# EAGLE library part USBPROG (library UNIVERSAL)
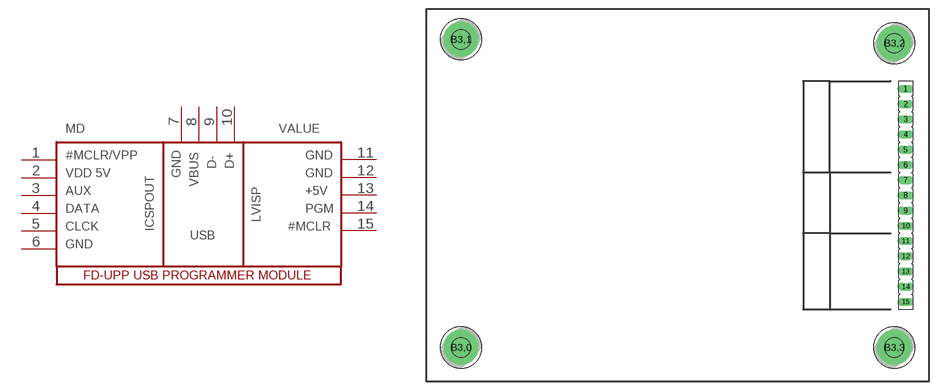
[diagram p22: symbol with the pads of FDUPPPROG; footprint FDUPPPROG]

Designator prefix MD

## USBPROG  [FDUPPPROG]
1  1
2  2
3  3
4  4
5  5
6  6
7  7
8  8
9  9
10  10
11  11
12  12
13  13
14  14
15  15

## Footprint FDUPPPROG (pad centres in mm)
Modul programatora ICD2 Microchip.
drill 0.813 long: 1 80.01,48.895; 2 80.01,46.355; 3 80.01,43.815; 4 80.01,41.275; 5 80.01,38.735; 6 80.01,36.195; 7 80.01,33.655; 8 80.01,31.115; 9 80.01,28.575; 10 80.01,26.035; 11 80.01,23.495; 12 80.01,20.955; 13 80.01,18.415; 14 80.01,15.875; 15 80.01,13.335
drill 3 pad 5.842: B3,0 5.715,5.715; B3,1 5.715,57.15; B3,2 78.105,56.515; B3,3 78.105,5.715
